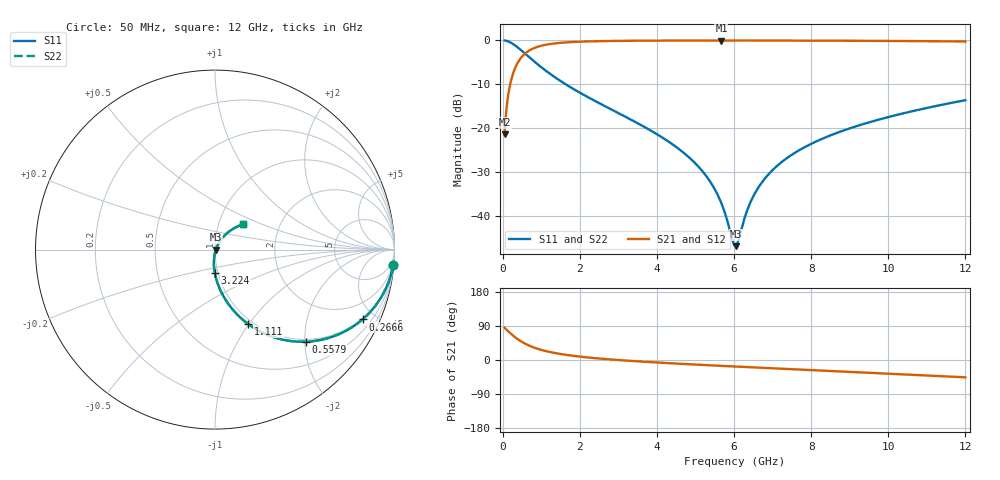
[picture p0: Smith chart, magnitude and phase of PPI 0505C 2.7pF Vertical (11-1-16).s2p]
# GHz S MA R 50
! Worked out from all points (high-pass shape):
!   1601 points, 50 MHz to 12 GHz, reference 50 ohm
!   highest |S21| = -0.04 dB at 5.674 GHz (marker M1); lowest = -21.4 dB at 50 MHz (marker M2)
!   |S21| within 3 dB of the highest: 576.3 MHz to end of sweep
!   lowest |S11| = -46.8 dB at 6.04 GHz (marker M3), VSWR 1.01, Z = 50.4 - j0.131 ohm
!   |S11| at or under -10 dB: 1.634 GHz to end of sweep
!   |S22| runs from -46.8 to 0.0 dB; largest |S21 - S12| = 0
!   S11 on the Smith chart (normalised r, x): 50 MHz: 1, -23; 266.6 MHz: 0.95, -4.25; 557.9 MHz: 0.95, -2.02; 1.111 GHz: 0.95, -0.99; 3.224 GHz: 0.96, -0.26; 12 GHz: 1.30, +0.38
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0.05  0.9963 -5.0  0.08528 85.0  0.08528 85.0  0.9963 -5.0
0.1620312  0.9635 -16.0  0.2674 74.0  0.2674 74.0  0.9635 -16.0
0.2665938  0.9093 -25.3  0.4156 64.6  0.4156 64.6  0.9093 -25.3
0.4010313  0.823 -35.7  0.5671 54.2  0.5671 54.2  0.823 -35.7
0.557875  0.72 -45.5  0.6927 44.4  0.6927 44.4  0.72 -45.5
0.8118125  0.5771 -56.9  0.815 32.9  0.815 32.9  0.5771 -56.9
1.110562  0.4537 -66.0  0.8891 23.8  0.8891 23.8  0.4537 -66.0
2.044156  0.2478 -80.9  0.966 8.4  0.966 8.4  0.2478 -80.9
3.224219  0.1323 -90.2  0.9877 -1.7  0.9877 -1.7  0.1323 -90.2
4.038312  0.08366 -94.3  0.9925 -6.8  0.9925 -6.8  0.08366 -94.3
5.069  0.03693 -96.0  0.9948 -12.4  0.9948 -12.4  0.03693 -96.0
5.412562  0.02352 -93.7  0.9951 -14.2  0.9951 -14.2  0.02352 -93.7
5.673969  0.01396 -87.1  0.9951 -15.5  0.9951 -15.5  0.01396 -87.1
6.025  0.004584 -23.1  0.9951 -17.2  0.9951 -17.2  0.004584 -23.1
6.039937  0.004567 -16.5  0.995 -17.3  0.995 -17.3  0.004567 -16.5
6.107156  0.005209 10.5  0.995 -17.6  0.995 -17.6  0.005209 10.5
6.413375  0.014 51.2  0.9948 -19.1  0.9948 -19.1  0.014 51.2
6.742  0.02491 58.1  0.9944 -20.7  0.9944 -20.7  0.02491 58.1
7.272281  0.04253 60.0  0.9935 -23.2  0.9935 -23.2  0.04253 60.0
8.019156  0.06715 58.7  0.9918 -26.6  0.9918 -26.6  0.06715 58.7
10.01331  0.1346 51.3  0.9839 -36.0  0.9839 -36.0  0.1346 51.3
12  0.2087 42.3  0.9698 -45.7  0.9698 -45.7  0.2087 42.3
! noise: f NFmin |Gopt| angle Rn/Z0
0.05  0.0007406  0.9383  1.776  0.002676
1.372  0.005716  0.7616  4.836  0.004854
2.701  0.00922  0.7163  8.362  0.006389
4.031  0.01234  0.6893  11.93  0.007643
5.36  0.01529  0.6712  15.49  0.008789
6.682  0.01815  0.6589  18.97  0.0099
8.012  0.02104  0.6508  22.43  0.01104
9.341  0.02398  0.6462  25.82  0.01224
10.67  0.02704  0.6446  29.15  0.01354
12  0.03026  0.6455  32.42  0.01497
